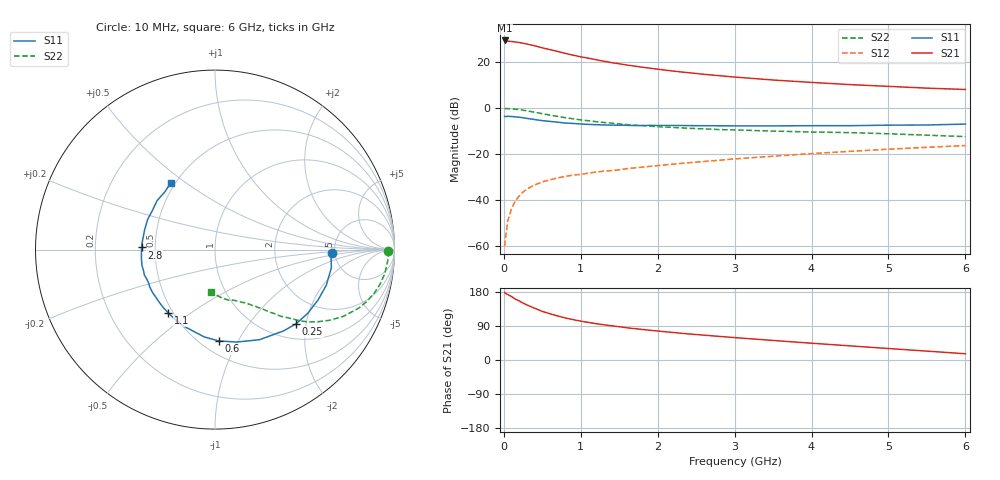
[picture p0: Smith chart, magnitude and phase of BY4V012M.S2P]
! SIEMENS Small Signal Semiconductors
! BFY420
! Si NPN RF SIEGET Grounded Emitter Transistor in MICRO-X
! VCE = 4 V  IC = 12 mA
! Common Emitter S-Parameters:  October  1996
# GHz  S  MA  R  50
!  f  S11  S21  S12  S22
! GHz  MAG  ANG  MAG  ANG  MAG  ANG  MAG  ANG
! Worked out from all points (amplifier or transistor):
!   36 points, 10 MHz to 6 GHz, reference 50 ohm
!   highest |S21| = 29.3 dB at 10 MHz (marker M1)
!   |S21| within 3 dB of that: start of sweep to 477.1 MHz
!   unconditionally stable (mu >= 1): start of sweep to 16.46 MHz; 2.394 GHz to end of sweep
!   at 250 MHz: K = 0.27, MSG = 32.3 dB, |S12| = -36.5 dB
!   at 1.4 GHz: K = 0.80, MSG = 23.4 dB, |S12| = -27.2 dB
!   at 6 GHz: K = 1.08, MAG = 10.5 dB, |S12| = -16.3 dB
!   S11 on the Smith chart (normalised r, x): 10 MHz: 4.72, -0.36; 250 MHz: 1.32, -1.75; 600 MHz: 0.61, -0.84; 1.1 GHz: 0.47, -0.41; 2.8 GHz: 0.42, +0.01; 6 GHz: 0.47, +0.44
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0.01  0.6521 -1.9  29.09 178.6  0.001 39.4  0.9631 -0.5
0.02  0.6479 -3.3  28.75 176.1  0.0014 46.1  0.967 -1.4
0.1  0.6511 -17.8  27.6 167.5  0.0065 76.1  0.9559 -8.0
0.15  0.6392 -25.9  26.95 160.6  0.0096 71.1  0.9386 -12.0
0.2  0.6272 -34.4  26.25 155.9  0.0123 72.4  0.9184 -15.5
0.25  0.6123 -42.5  25.34 150.2  0.015 68.1  0.8913 -19.1
0.3  0.5924 -49.9  24.34 145.1  0.0174 67.0  0.8655 -22.1
0.4  0.5599 -63.7  22.31 136.7  0.0213 62.6  0.8059 -27.5
0.5  0.5293 -76.6  20.11 128.3  0.0248 59.9  0.7496 -31.7
0.6  0.5095 -87.6  18.38 122.0  0.0275 56.6  0.699 -35.1
0.7  0.49 -97.1  16.78 116.1  0.0302 55.9  0.6543 -38.0
0.8  0.4689 -105.7  15.23 111.0  0.0327 53.6  0.6135 -40.2
0.9  0.46 -112.9  13.94 106.5  0.0348 53.2  0.5792 -41.8
1.1  0.4387 -126.2  11.96 99.2  0.0384 52.8  0.5257 -45.1
1.3  0.427 -137.0  10.31 93.0  0.0423 52.9  0.4832 -47.3
1.6  0.4192 -150.0  8.514 85.0  0.0481 52.7  0.4352 -50.6
2.2  0.4162 -168.1  6.295 72.6  0.0603 52.0  0.3774 -56.0
2.8  0.4093 178.3  5.001 62.3  0.0732 50.6  0.3387 -60.8
3.5  0.4071 164.5  4.03 51.6  0.0895 47.6  0.3138 -66.2
4.5  0.4115 147.8  3.206 37.3  0.1141 41.2  0.2911 -75.0
5.5  0.4262 130.9  2.686 23.4  0.1397 33.6  0.256 -87.1
6  0.4457 123.6  2.512 16.5  0.1524 29.3  0.2385 -94.9
